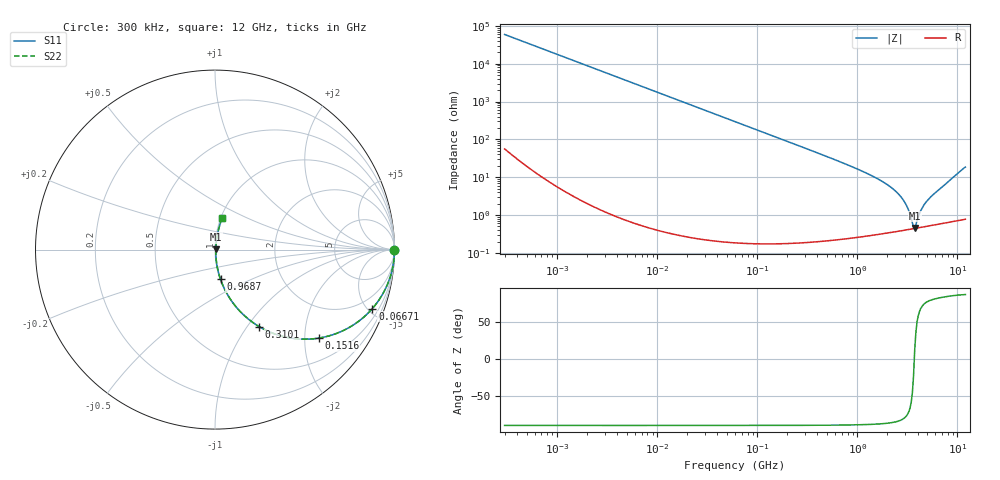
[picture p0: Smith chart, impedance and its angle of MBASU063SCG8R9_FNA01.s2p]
! MBASU063SCG8R9_FNA01  S-PARAMETER MODEL  ( General Type )
! Model Generated by TAIYO YUDEN Corporation (http://www.ty-top.com)
! Version 1.0
! TAIYO YUDEN Control No. 130801
! Copyright(c) 2013 TAIYO YUDEN CO.,LTD. All Rights Reserved.
! Product Description (link to TY-COMPAS)
! https://ds.yuden.co.jp/TYCOMPAS/or/detail?pn=MBASU063SCG8R9DFNA01&u=M
! Products Name : Multilayer Ceramic Capacitors
! Characteristics :
!  Capacitance : 8.9 pF , Rated Voltage : 50V , TCC : CG / C0G
!  Case Size : 0.6 x 0.3 / 0.024 x 0.012 [mm/inch] , Thickness : 0.3 / 0.012 [mm/inch]
!  (Conditions: Temperature = 25 degC , DC Bias Current/Voltage = 0A / 0V)
! External Node Assignments :
!  1  o---| |---o  2
! GND o---------o GND
! Frequency Range : 0.3MHz  -  12000MHz  [ 401 STEP ]
# MHz S RI R 50
! Freq[MHz].  S11 Real  S11 Imag  S21 Real  S21 Imag  S12 Real  S12 Imag  S22 Real  S22 Imag
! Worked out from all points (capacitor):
!   401 points, 300 kHz to 12 GHz, reference 50 ohm
!   read as one part in series: C = 8.94 pF near 316.3 kHz
!   lowest |Z| = 453 mohm at 3.741 GHz (marker M1)
!   series resonance near 3.707 GHz, so ESL is about 210 pH
!   S11 on the Smith chart (normalised r, x): 300 kHz: open; 66.71 MHz: 1.00, -5.33; 151.6 MHz: 1.00, -2.34; 310.1 MHz: 1.00, -1.14; 968.7 MHz: 1.01, -0.34; 12 GHz: 1.02, +0.37
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0.3  1 -0.00169  4.43e-06 0.00169  4.43e-06 0.00169  1 -0.00169
1.769972  0.9999 -0.00994  0.000101 0.00994  0.000101 0.00994  0.9999 -0.00994
10.44266  0.9966 -0.0585  0.00344 0.0585  0.00344 0.0585  0.9966 -0.0585
26.39317  0.9784 -0.1451  0.0216 0.1451  0.0216 0.1451  0.9784 -0.1451
60  0.8978 -0.3027  0.1022 0.3027  0.1022 0.3027  0.8978 -0.3027
66.70707  0.8766 -0.3286  0.1234 0.3286  0.1234 0.3286  0.8766 -0.3286
151.6462  0.5785 -0.4931  0.4215 0.4931  0.4215 0.4931  0.5785 -0.4931
310.0777  0.2459 -0.429  0.7541 0.429  0.7541 0.429  0.2459 -0.429
353.9943  0.1998 -0.3979  0.8002 0.3979  0.8002 0.3979  0.1998 -0.3979
555.3718  0.091 -0.2842  0.909 0.2842  0.909 0.2842  0.091 -0.2842
968.706  0.0308 -0.1655  0.9692 0.1655  0.9692 0.1655  0.0308 -0.1655
1519.776  0.0123 -0.096  0.9877 0.096  0.9877 0.096  0.0123 -0.096
2088.533  0.00676 -0.0577  0.9932 0.0577  0.9932 0.0577  0.00676 -0.0577
2514.07  0.00514 -0.038  0.9949 0.038  0.9949 0.038  0.00514 -0.038
2870.14  0.00453 -0.0247  0.9955 0.0247  0.9955 0.0247  0.00453 -0.0247
3190.978  0.00431 -0.0145  0.9957 0.0145  0.9957 0.0145  0.00431 -0.0145
3547.679  0.00432 -0.00433  0.9957 0.00433  0.9957 0.00433  0.00432 -0.00433
3740.715  0.00441 0.00096  0.9956 -0.00096  0.9956 -0.00096  0.00441 0.00096
3841.137  0.00447 0.00318  0.9955 -0.00318  0.9955 -0.00318  0.00447 0.00318
4502.883  0.00505 0.0155  0.995 -0.0155  0.995 -0.0155  0.00505 0.0155
5140.631  0.00576 0.0254  0.9942 -0.0254  0.9942 -0.0254  0.00576 0.0254
12000  0.04 0.1761  0.96 -0.1761  0.96 -0.1761  0.04 0.1761
